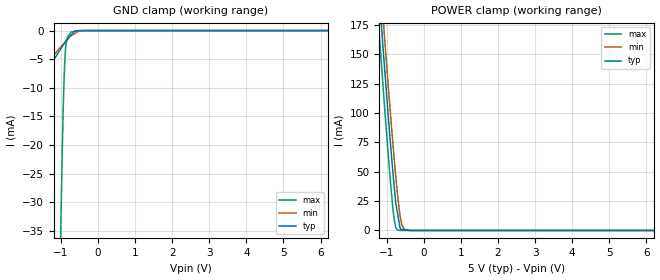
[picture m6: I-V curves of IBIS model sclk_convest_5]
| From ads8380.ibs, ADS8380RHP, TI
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|   sclk_convest_5 Model
[Model]   sclk_convest_5
Model_type   Input
Vinl = 0.8
Vinh = 4
|   typ   min   max
|   (nom PVT)   (fast PVT)   (slow PVT)
|C_comp from frequency sweep method (F=40MHz)
|Average
C_comp   8.045e-13   7.845e-13   8.268e-13
|C_comp from LC tank measurement(L=1nH)
|Average
|Resonant Frequency(Hz)   6.880e+09   7.170e+09   6.610e+09
|C_comp   5.357e-13   4.932e-13   5.803e-13
| Where nom  PVT is Nominal Process, 5V, 35C
|   Fast PVT is Strong Process,  5.25V, -40C
|   Slow PVT is Weak Process,   4.75V, 95C
[Model Spec]
Vinl   0.8   0.8   0.8
Vinh   4.0   3.75   4.25
[Voltage Range]   5   4.75   5.25
|Ambient Temperature   25   85   -40
|Junction Temperature
[Temperature Range]   35   95   -40
[Power Clamp Reference]   5   4.75   5.25
[GND Clamp Reference]   0   0   0
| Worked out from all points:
|   GND clamp passes 1 mA (typ) near -0.76 V on its own axis
|   POWER clamp passes 1 mA (typ) near -0.62 V on its own axis
[GND Clamp]
|   Voltage   I(typ)   I(min)   I(max)
-5V       -51.14mA   -37.96mA   -1.888A
-4.75V    -47.95mA   -35.65mA   -1.771A
-4.21V    -41.13mA   -30.65mA   -1.516A
-3.533V   -32.56mA   -24.38mA   -1.198A
-2.67V    -21.64mA   -16.53mA   -792.8mA
-1.008V   -3.206mA   -2.891mA   -36.15mA
-939.7mV  -2.519mA   -2.392mA   -14.05mA
-892.5mV  -2.043mA   -2.046mA   -4.874mA
-829.5mV  -1.508mA   -1.585mA   -1.265mA
-729.8mV  -784.8uA   -924.3uA   -289.8uA
-503.5mV  -20.08uA   -23.98uA   -21.48uA
10V       0A         0A         0A
[POWER Clamp]
|   Voltage   I(typ)   I(min)   I(max)
-5V       1.905A     1.922A     1.884A
-1.302V   242mA      267.3mA    209.7mA
-1.126V   166.8mA    192.3mA    134.1mA
-1.08V    147.2mA    173.1mA    114.4mA
-955.5mV  95.9mA     121.9mA    62.77mA
-834.7mV  49.93mA    74.38mA    18.9mA
-761.2mV  24.49mA    47.49mA    2.961mA
-698.3mV  12.62mA    27.18mA    218.3uA
-640mV    1.834mA    12.45mA    14.73uA
-598.5mV  870.6uA    5.545mA    1.881uA
-356.3mV  494.1nA    6.232uA    1.12uA
10V       0A         0A         0A
